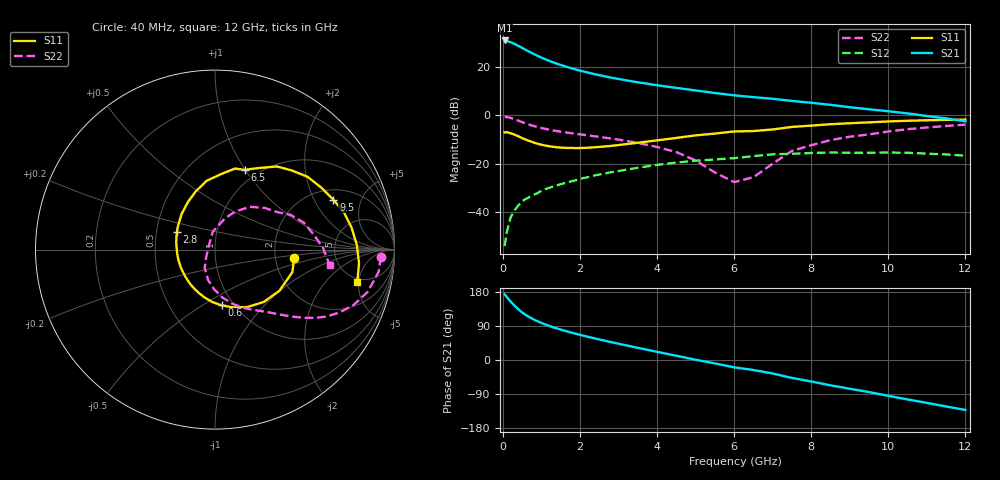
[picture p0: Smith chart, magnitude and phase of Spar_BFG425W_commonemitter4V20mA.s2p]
! Filename: 420bfg425.001
! BFG425W Field C1
! V1=8.380E-001V,V2=4.000E+000V, I1=2.416E-004A, I2=2.001E-002A
# GHz  S  MA  R 50
!  S11  S21  S12  S22
!Freq(GHz)  Mag  Ang  Mag  Ang  Mag  Ang  Mag  Ang
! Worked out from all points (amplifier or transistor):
!   44 points, 40 MHz to 12 GHz, reference 50 ohm
!   highest |S21| = 30.9 dB at 40 MHz (marker M1)
!   |S21| within 3 dB of that: start of sweep to 486.6 MHz
!   unconditionally stable (mu >= 1): start of sweep to 45.07 MHz; 1.39 GHz to end of sweep
!   at 700 MHz: K = 0.76, MSG = 29.8 dB, |S12| = -33.6 dB
!   at 2.4 GHz: K = 1.14, MAG = 18.6 dB, |S12| = -24.7 dB
!   at 12 GHz: K = 1.35, MAG = 3.6 dB, |S12| = -16.7 dB
!   S11 on the Smith chart (normalised r, x): 40 MHz: 2.56, -0.28; 600 MHz: 0.88, -0.61; 2.8 GHz: 0.64, +0.14; 6.5 GHz: 0.87, +0.99; 9.5 GHz: 2.52, +2.88; 12 GHz: 4.53, -4.78
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0.04  0.444 -5.7  35.02 173.2  0.002 57.3  0.925 -2.5
0.1  0.449 -16.3  34.01 166.0  0.004 74.4  0.92 -7.7
0.2  0.426 -32.5  32.15 153.8  0.008 72.2  0.883 -15.4
0.3  0.399 -46.8  29.62 143.2  0.011 69.5  0.831 -21.9
0.4  0.368 -60.4  26.99 133.7  0.014 66.7  0.775 -27.0
0.5  0.338 -72.5  24.46 125.2  0.017 63.8  0.723 -31.1
0.6  0.313 -83.2  22.13 118.2  0.019 62.5  0.676 -34.2
0.7  0.293 -92.7  20.1 112.3  0.021 61.1  0.635 -36.8
0.9  0.259 -109.7  16.79 102.0  0.025 59.5  0.572 -40.8
1  0.247 -117.3  15.46 97.6  0.028 58.9  0.547 -42.4
1.2  0.23 -130.8  13.29 89.9  0.032 57.7  0.506 -45.5
1.6  0.214 -154.3  10.29 77.2  0.04 55.2  0.447 -50.9
2.2  0.214 177.5  7.618 61.4  0.053 50.0  0.386 -59.5
2.8  0.234 154.7  6.01 47.3  0.067 43.5  0.332 -69.0
3.5  0.272 133.1  4.797 32.1  0.083 34.6  0.27 -81.2
4.5  0.342 108.2  3.677 11.2  0.106 20.2  0.174 -102.7
5.5  0.42 85.9  2.883 -9.0  0.123 4.7  0.066 -138.6
6.5  0.474 69.6  2.371 -26.4  0.144 -7.3  0.053 121.6
8.5  0.656 38.2  1.643 -66.8  0.171 -44.3  0.308 50.7
9.5  0.716 22.9  1.33 -84.6  0.169 -61.2  0.404 31.2
10.5  0.771 9.0  1.095 -104.1  0.169 -79.8  0.518 16.8
12  0.813 -12.7  0.751 -131.7  0.147 -110.0  0.644 -7.7
